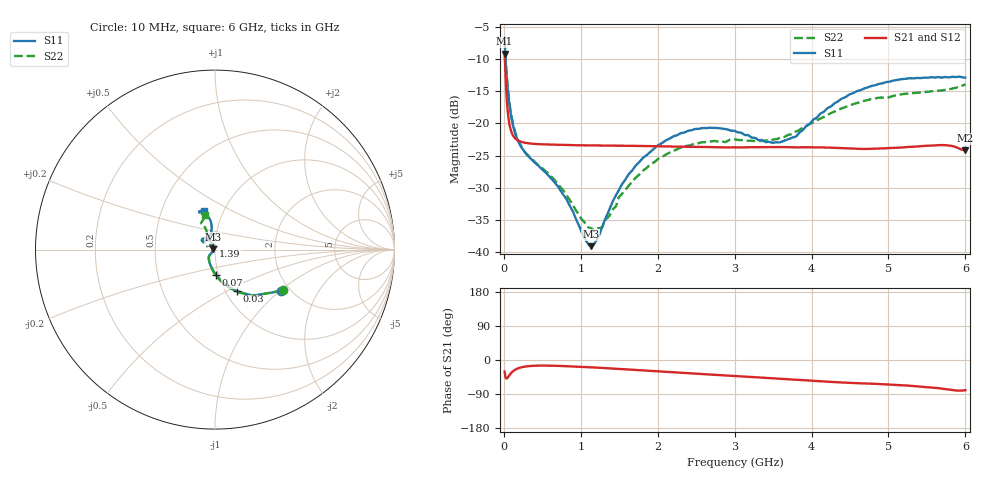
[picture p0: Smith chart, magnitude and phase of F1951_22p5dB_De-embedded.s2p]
! Integrated Device Technology
! Corporate Headquarters
! 6024 Silver Creek Valley Road
! San Jose, CA 95138  USA
! Phone:  1-408-284-8200
! Toll Free:  1-800-223-1366
! Webpage:  http://www.idt.com/
! Timing and RF Division
! 515 Groton Road, Suite 102
! Westford, MA 01886-6024
! Device:  F1951
! Description: 6-bit 0.5 dB Digital Step Attenuator
! Frequency:  100.0 -  4000.00 MHz
! Package:  4x4 mm Thin QFN Plastic Package: 24 pin
! Ports:  2 RF, 6 DC
!  Pin  1  = NC
!  Pin  2  = RF1  =  Port 1
!  Pin  3  = GND
!  Pin  4  = NC
!  Pin  5  = Serial Data Out (SDO)
!  Pin  6  = NC
!  Pin  7  = Reset Bar ( RSTb)
!  Pin  8  = Clock (CLK)
!  Pin  9  = Chip Select Bar (CSb)
!  Pin 10  = NC
!  Pin 11  = Serial Data In (SDI)
!  Pin 12  = NC
!  Pin 13  = NC
!  Pin 14  = VDD
!  Pin 15  = NC
!  Pin 16  = GND
!  Pin 17  = RF2  =  Port 2
!  Pin 18  = NC
!  Pin 19  = GND
!  Pin 20  = GND
!  Pin 21  = GND
!  Pin 22  = GND
!  Pin 23  = GND
!  Pin 24  = GND
! State:  45
! Atten State:  22.5 dB
! Voltage:  +3.30 Volts
! Current:  0.488 mA
! Data:  The device was measured on a F195X evaluation board which has
!  individual transmission lines to the RF pins.  Data was collected
!  de-embedded using a Automatic Fixture Removal [AFR] (Keysight Technologies).
!  The reference plane is the edge of the package pin.
! Misc:  Lot Code  1225BCA
!  Action Tracker AT0399
! Date Measured:  2018-09-13
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# GHz S dB R 50
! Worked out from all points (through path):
!   600 points, 10 MHz to 6 GHz, reference 50 ohm
!   highest |S21| = -9.19 dB at 10 MHz (marker M1); lowest = -24.2 dB at 6 GHz (marker M2)
!   group delay of S21, straight-line fit = 30.3 ps
!   lowest |S11| = -39.0 dB at 1.13 GHz (marker M3), VSWR 1.02, Z = 48.9 + j0.139 ohm
!   |S11| at or under -10 dB: 21.97 MHz to end of sweep
!   |S22| runs from -36.7 to -7.1 dB; largest |S21 - S12| = 0.0002
!   S11 on the Smith chart (normalised r, x): 10 MHz: 1.79, -1.02; 30 MHz: 1.13, -0.56; 70 MHz: 0.97, -0.28; 1.39 GHz: 0.98, +0.04; 6 GHz: 0.81, +0.37
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0.01  -7.26 -32.3  -9.19 -30.5  -9.19 -30.5  -7.14 -30.9
0.03  -11.62 -62.3  -14.67 -48.7  -14.67 -48.7  -11.28 -61.1
0.07  -16.87 -87.1  -19.96 -40.8  -19.96 -40.8  -16.56 -86.6
0.14  -21.27 -108.3  -22.23 -26.6  -22.22 -26.6  -21.03 -107.3
0.24  -23.92 -122.5  -22.91 -18.7  -22.91 -18.7  -23.83 -122.0
0.7  -29.73 -134.6  -23.31 -15.4  -23.31 -15.5  -29.35 -137.2
0.85  -32.59 -138.3  -23.36 -16.7  -23.36 -16.7  -31.74 -141.5
1.01  -36.82 -154.1  -23.41 -18.2  -23.41 -18.2  -34.84 -151.6
1.13  -39.04 172.7  -23.42 -19.2  -23.42 -19.2  -36.22 -169.1
1.26  -36.70 134.7  -23.43 -20.7  -23.43 -20.7  -36.20 165.6
1.39  -32.84 119.7  -23.45 -22.2  -23.44 -22.2  -33.97 146.0
1.63  -27.79 116.4  -23.48 -25.1  -23.48 -25.1  -29.58 133.4
2.01  -23.37 123.8  -23.55 -30.0  -23.55 -30.0  -25.47 134.9
2.49  -20.86 136.7  -23.64 -36.1  -23.64 -36.1  -23.15 142.3
3.01  -21.21 146.5  -23.72 -42.5  -23.72 -42.4  -22.49 145.8
3.58  -22.96 125.3  -23.68 -49.4  -23.68 -49.4  -22.27 128.6
3.79  -22.08 109.7  -23.73 -52.1  -23.73 -52.0  -21.30 121.7
4.01  -19.60 101.1  -23.71 -54.8  -23.71 -54.7  -19.93 116.3
4.49  -15.53 99.1  -23.88 -60.3  -23.88 -60.3  -17.24 114.5
5.01  -13.54 107.7  -23.83 -64.6  -23.83 -64.6  -15.94 117.1
5.72  -12.83 112.4  -23.36 -76.2  -23.36 -76.2  -14.83 110.2
6  -12.90 106.1  -24.19 -79.8  -24.19 -79.7  -13.95 106.3
